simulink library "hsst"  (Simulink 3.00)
undefined symbols (not defined in the file or in its folder): Final, l, m3, s, to
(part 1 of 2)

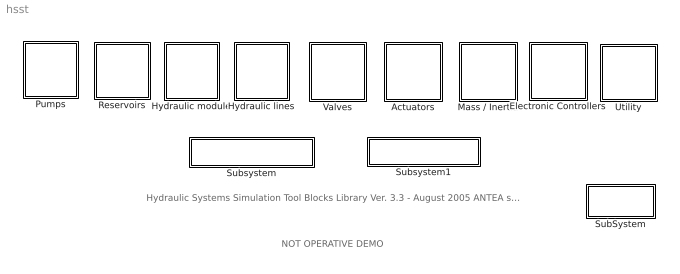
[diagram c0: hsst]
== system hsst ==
  note: Hydraulic Systems Simulation Tool Blocks Library Ver. 3.3 - August 2005 ANTEA s.a.s.
  note: NOT OPERATIVE DEMO
  Actuators : Subsystem
  Electronic Controllers : Subsystem
  Hydraulic lines : Subsystem
  Hydraulic module : Subsystem
  Mass / Inertia : Subsystem
  Pumps : Subsystem
  Reservoirs : Subsystem
  SubSystem : Subsystem
  Subsystem : Subsystem  StartFcn=Start_r
  Subsystem1 : Subsystem
  Utility : Subsystem
  Valves : Subsystem

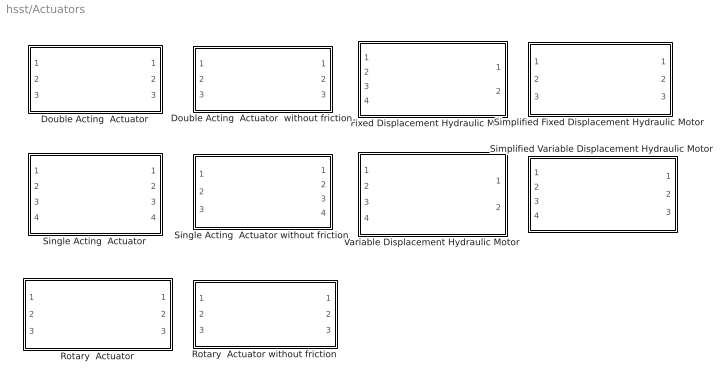
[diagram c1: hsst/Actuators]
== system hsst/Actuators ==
  Double Acting  Actuator : Subsystem  mask{Ai=, Au=, X_s=[0 0], m=, V0_out=1e-15, V0_in=1e-15, F0=, K=, C=, c_leak=, Fs=, Fd=}
      mask prompts: Ai "Piston Input Area [m2]"; Au "Piston Output Area [m2]"; X_s "Piston Maximum Stroke [m]"; m "Piston Mass [kg]"; V0_out "Piston Outlet Lost Volume [m3]"; V0_in "Piston Inlet Lost Volume [m3]"; F0 "Piston Spring Preload [N]"; K "Piston Spring Stiffness [N/m]"; C "Piston Damping [N/(m/s)]"; c_leak "Piston leakage coefficient [(m3/s)/sqr(Pa)]"; Fs "Static Friction Force [N]"; Fd "Dynamic Friction Force [N]"
      mask init:
      | global beta
  Double Acting  Actuator  without friction : Subsystem  mask{Ai=, Au=, X_s=[0 0], m=, V0_out=1.e-15, V0_in=1.e-15, F0=0, K=0, C=0}
      mask prompts: Ai "Piston Input Area [m2]"; Au "Piston Output Area [m2]"; X_s "Piston Maximum Stroke [m]"; m "Piston Mass [kg]"; V0_out "Piston Outlet Lost Volume [m3]"; V0_in "Piston Inlet Lost Volume [m3]"; F0 "Piston Spring Preload [N]"; K "Piston Spring Stiffness [N/m]"; C "Piston Damping [N/(m/s)]"
      mask init:
      | global beta
  Fixed Displacement Hydraulic Motor : Subsystem  mask(Hydraulic motor){Ds=0, Im=0, V0_out=0, Cm=0, cfug=0, c_leak=0, Ploss=0, Cf=0, rkm=0, Ts=0, Td=0}
      mask prompts: Ds "Displacement [cc/rev]"; Im "Total Motor Inertia [kg*m2]"; V0_out "Hydraulic line volume [m3]"; Cm "Actuator Internal Damping [Nm/(rad/s)]"; cfug "Interport Leakage coeff. [(m3/s)/Pa]"; c_leak "Case Drain Leakage Coef. [(m3/s)/Pa]"; Ploss "Ploss (Help for definition)"; Cf "Cf (Help for definition)"; rkm "rkm (Help for definition)"; Ts "Static FrictionTorque [Nm]"; Td "Dynamic Friction Torque [Nm]"
      mask init:
      | global beta
      | D = Ds/1e6;
      | V0_in = V0_out;
  Rotary  Actuator : Subsystem  mask(Rotary Actuator){Air=0, X_s=[0 0], m=0, V0_out=1e-15, F0=0, K=0, C=0, c_leak=0, Fs=0, Fd=0}
      mask prompts: Air "Displacement [cc/rev]"; X_s "Actuator Maximum Stroke [rad]"; m "Total Actuator Inertia [kg*m2]"; V0_out "Minimum Hydraulic Volume [m3]"; F0 "Actuator Spring Preload [Nm]"; K "Actuator Spring Stiffness [Nm/rad]"; C "Actuator Internal Damping [Nm/(rad/s)]"; c_leak "Actuator Internal Leakage Coefficient [(m3/s)/sqr(Pa)]"; Fs "Static Friction Force [N]"; Fd "Dynamic Friction Force [N]"
      mask init:
      | global beta
      | 
      | Ai = Air*1.e-6/6.2831853;
      | V0_in = V0_out;
      | Au = Ai;
  Rotary  Actuator without friction : Subsystem  mask(Rotary Actuator){Air=0, X_s=[0 0], m=0, V0_out=1e-15, F0=0, K=0, C=0}
      mask prompts: Air "Displacement [cc/rev]"; X_s "Actuator Maximum Stroke [rad]"; m "Total Actuator Inertia [kg*m2]"; V0_out "Minimum Hydraulic Volume [m3]"; F0 "Actuator Spring Preload [Nm]"; K "Actuator Spring Stiffness [Nm/rad]"; C "Actuator Internal Damping [Nm/(rad/s)]"
      mask init:
      | global beta
      | 
      | Ai = Air*1.e-6/6.2831853;
      | V0_in = V0_out;
      | Au = Ai;
  Simplified Fixed Displacement Hydraulic Motor : Subsystem  mask(Hydraulic motor){Ds=0, Im=0, V0_out=0, Cm=0, etav=0, etam=0}
      mask prompts: Ds "Displacement [cc/rev]"; Im "Total Motor Inertia [kg*m2]"; V0_out "Hydraulic line volume [m3]"; Cm "Actuator Internal Damping [Nm/(rad/s)]"; etav "Volumetric efficiency [-]"; etam "Mechanical  efficiency [-]"
      mask init:
      | global beta
      | D = Ds/1e6;
      | V0_in = V0_out;
  Simplified Variable Displacement Hydraulic Motor : Subsystem  mask(Variable diplacement hydraulic motor ){Ds_mx=0, Ds_mn=0, Im=0, V0_out=0, Cm=0, etav=0, etam=0}
      mask prompts: Ds_mx "Maximum Displacement [cc/rev]"; Ds_mn "Minimum Displacement [cc/rev]"; Im "Total Motor Inertia [kg*m2]"; V0_out "Hydraulic line volume [m3]"; Cm "Actuator Internal Damping [Nm/(rad/s)]"; etav "Volumetric efficiency [-]"; etam "Mechanical  efficiency [-]"
      mask init:
      | global beta
      | D_mx = Ds_mx/1e6;
      | D_mn = Ds_mn/1e6;
      | V0_in = V0_out;
  Single Acting  Actuator : Subsystem  mask(Single Acting Actuator){Ai=, Au=, X_s=[ ], m=, V0_in=1e-15, V0_out=1e-15, F0=, K=, C=, Fd=, Fs=}
      mask prompts: Ai "Piston Controlled Pressure Area [m2]"; Au "Piston Uncontrolled pressure Area [m2]"; X_s "Piston Maximum Stroke [m]"; m "Total Connected Mass [kg]"; V0_in "Piston Controlled Side Lost Volume [m3]"; V0_out "Piston Uncontrolled Side Lost Volume [m3]"; F0 "Piston Spring Preload [N]"; K "Piston Spring Stiffness [N/m]"; C "Piston Damping [N/(m/s)]"; Fd "Dyn. friction"; Fs "Static friction"
      mask init:
      | global beta
  Single Acting  Actuator without friction : Subsystem  mask(Single Acting Actuator){Ai=, Au=, X_s=[ ], m=, V0_in=1e-15, V0_out=1e-15, F0=, K=, C=}
      mask prompts: Ai "Piston Controlled Pressure Area [m2]"; Au "Piston Uncontrolled pressure Area [m2]"; X_s "Piston Maximum Stroke [m]"; m "Total Connected Mass [kg]"; V0_in "Piston Controlled Side Lost Volume [m3]"; V0_out "Piston Uncontrolled Side Lost Volume [m3]"; F0 "Piston Spring Preload [N]"; K "Piston Spring Stiffness [N/m]"; C "Piston Damping [N/(m/s)]"
      mask init:
      | global beta
  Variable Displacement Hydraulic Motor : Subsystem  mask(Variable diplacement hydraulic motor ){Ds_mx=0, Ds_mn=0, Im=0, V0_out=0, Cm=0, cfug=0, c_leak=0, Ploss=0, Cf=0, rkm=0, Ts=0, Td=0}
      mask prompts: Ds_mx "Maximum Displacement [cc/rev]"; Ds_mn "Minimum Displacement [cc/rev]"; Im "Total Motor Inertia [kg*m2]"; V0_out "Hydraulic line volume [m3]"; Cm "Actuator Internal Damping [Nm/(rad/s)]"; cfug "Interport Leakage coeff. [(m3/s)/Pa]"; c_leak "Case Drain Leakage Coef. [(m3/s)/Pa]"; Ploss "Ploss (Help for definition)"; Cf "Cf (Help for definition)"; rkm "rkm (Help for definition)"; Ts "Static FrictionTorque [Nm]"; Td "Dynamic Friction Torque [Nm]"
      mask init:
      | global beta
      | D_mx = Ds_mx/1e6;
      | D_mn = Ds_mn/1e6;
      | V0_in = V0_out;

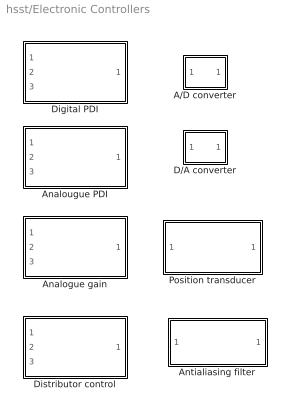
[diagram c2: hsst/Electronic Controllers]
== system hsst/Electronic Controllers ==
  A/D converter : Subsystem  mask(A/D){n_bit=, n_max=}
      mask prompts: n_bit "Number of bit (excluding the sign bit: saturation = +/- n° bit)"; n_max "Satuaration value  (output saturation at +/- this value)"
      mask init:
      | lsb=n_max/2^n_bit;
  Analogue gain : Subsystem  mask(Analog controller){Gp=, H=, p_opm=}
      mask prompts: Gp "Proportional gain"; H "Feedback gain"; p_opm "Minimum Operative Pressure [MPa]"
      mask init:
      | p_op=p_opm*1.e6;
  Analougue PDI : Subsystem  mask(Analuogue PDI controller){Gp=[ ], Gi=[ ], Gd=[ ], tau=, Ls=[ ], Ls_1=[-Inf Inf], i_i_max=[-Inf Inf], H=, p_opm=, max_cp=Inf, max_cm=-Inf}
      mask prompts: Gp "Proportional gain (2 values: [- +])"; Gi "Integrative gain (2 values: [- +])"; Gd "Derivative gain (2 values: [- +])"; tau "First order filter constant [s]"; Ls "Integrator threshold (2 values)"; Ls_1 "Integrator band limit (2 values)"; i_i_max "Integrator current saturation [mA] (2 val)"; H "Feedback gain"; p_opm "Minimum Operative Pressure [MPa]"; max_cp "max curr"; max_cm "min curr"
      mask help: Digital PDI controller
      mask init:
      | % i_i_min=-i_i_max;
      | % Li=-Ls;
      | % Li_1=-Ls_1;
      | p_op=p_opm*1.e6;
  Antialiasing filter : Subsystem  mask(Antialiasing filter){fr=, zi=}
      mask prompts: fr "Undumped natural frequency [Hz]"; zi "Damping factor"
      mask init:
      | sig=2*pi*fr;
  D/A converter : Subsystem  mask(A/D){n_bit=, n_max=}
      mask prompts: n_bit "Number of bit (excluding the sign bit: saturation = +/- n° bit)"; n_max "Satuaration value  (output saturation at +/- this value)"
      mask init:
      | lsb=n_max/2^n_bit;
  Digital PDI : Subsystem  mask(PDI controller){Ts=, Tc=, Gp=[ ], Gi=[ ], Gd=[ ], tau=, Ls=[ ], Ls_1=[-Inf Inf], i_i_max=[-Inf Inf], H=, p_opm=, max_cp=Inf, max_cm=-Inf}
      mask prompts: Ts "Sampling time [s]"; Tc "Calculation time [s]"; Gp "Proportional gain (2 values: [- +])"; Gi "Integrative gain (2 values: [- +])"; Gd "Derivative gain (2 values: [- +])"; tau "First order filter constant [s]"; Ls "Integrator threshold (2 values)"; Ls_1 "Integrator band limit (2 values)"; i_i_max "Integrator current saturation [mA] (2 val)"; H "Feedback gain"; p_opm "Minimum Operative Pressure [MPa]"; max_cp "max curr"; max_cm "min curr"
      mask help: Digital PDI controller
      mask init:
      | % i_i_min=-i_i_max;
      | % Li=-Ls;
      | % Li_1=-Ls_1;
      | p_op=p_opm*1.e6;
  Distributor control : Subsystem  mask(Distributor controller){c_mx=, H=, p_opm=}
      mask prompts: c_mx "Maximum current"; H "Feedback gain"; p_opm "Minimum Operative Pressure [MPa]"
      mask init:
      | p_op=p_opm*1.e6;
  Position transducer : Subsystem  mask{bksl=}
      mask prompts: bksl "Position transducer backlash [actuator position unit]"

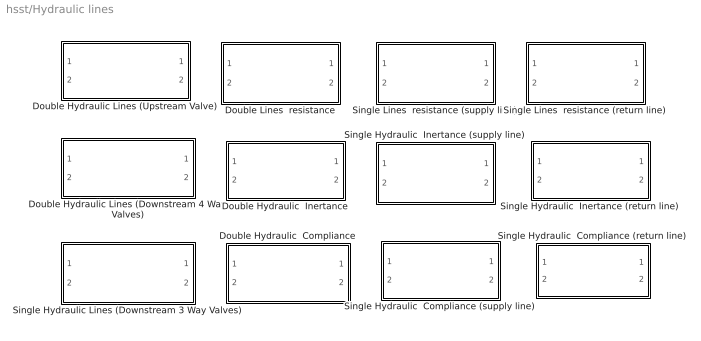
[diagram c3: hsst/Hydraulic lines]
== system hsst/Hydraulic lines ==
  Double Hydraulic  Compliance : Subsystem  mask(Double Hydraulic Compliance){C1=, C2=}
      mask prompts: C1 "Line 1 hydraulic compliance [m5/N]"; C2 "Line 2 hydraulic compliance [m5/N]"
  Double Hydraulic  Inertance : Subsystem  mask(Double Hydraulic Lines){rl1=, rl2=, rq1=, rq2=, L1=, L2=}
      mask prompts: rl1 "Line 1 linear resistance coefficient [Pa s/m3]"; rl2 "Line 2 linear resistance coefficient [Pa s/m3]"; rq1 "Line 1 quadratic resistance coefficient [Pa s2/m6]"; rq2 "Line 2 quadratic resistance coefficient [Pa s2/m6]"; L1 "Line 1 inertance [kg/m4]"; L2 "Line 2 inertance [kg/m4]"
  Double Hydraulic Lines (Downstream 4 Way Valves) : Subsystem  mask(Hydraulic Line){rl1=, rl2=, rq1=, rq2=, ll1=, ll2=, a1=, a2=}
      mask prompts: rl1 "Line 1 linear resistance coefficient [Pa s/m3]"; rl2 "Line 2 linear resistance coefficient [Pa s/m3]"; rq1 "Line 1 quadratic resistance coefficient [Pa s2/m6]"; rq2 "Line 2 quadratic resistance coefficient [Pa s2/m6]"; ll1 "Line 1 length [m]"; ll2 "Line 2  length [m]"; a1 "Line 1 section area [m2]"; a2 "Line 2 section area [m2]"
      mask init:
      | global rho
      | global beta
      | L1 = rho*ll1/a1;
      | L2 = rho*ll2/a2;
  Double Hydraulic Lines (Upstream Valve) : Subsystem  mask(Hydraulic Line){rl1=, rl2=, rq1=, rq2=, ll1=, ll2=, a1=, a2=}
      mask prompts: rl1 "Line 1 linear resistance coefficient [Pa s/m3]"; rl2 "Line 2 linear resistance coefficient [Pa s/m3]"; rq1 "Line 1 quadratic resistance coefficient [Pa s2/m6]"; rq2 "Line 2 quadratic resistance coefficient [Pa s2/m6]"; ll1 "Line 1 length [m]"; ll2 "Line 2  length [m]"; a1 "Line 1 section area [m2]"; a2 "Line 2 section area [m2]"
      mask init:
      | global rho
      | global beta
      | L1 = rho*ll1/a1;
      | L2 = rho*ll2/a2;
  Double Lines  resistance : Subsystem  mask(Lines resistance){rq1=, rl1=, rq2=, rl2=}
      mask prompts: rq1 "Line 1 quadratic resistance [Pa/(m6/s2)]"; rl1 "Line 1 linear resistance [Pa/(m3/s)]"; rq2 "Line 2 quadratic resistance [Pa/(m6/s2)]"; rl2 "Line 2 linear resistance [Pa/(m3/s)]"
      mask init:
      | global rho
      | global mu
      | q_min=.01/60000;
  Single Hydraulic  Compliance (return line) : Subsystem  mask(Single Hydraulic Compliance){C1=}
      mask prompts: C1 "Hydraulic compliance [m5/N]"
  Single Hydraulic  Compliance (supply line) : Subsystem  mask(Single Hydraulic Compliance){C1=}
      mask prompts: C1 "Hydraulic compliance [m5/N]"
  Single Hydraulic  Inertance (return line) : Subsystem  mask(Single Hydraulic Lines){rl1=, rq1=, L1=}
      mask prompts: rl1 "Linear resistance coefficient [Pa s/m3]"; rq1 "Quadratic resistance coefficient [Pa s2/m6]"; L1 "Inertance [kg/m4]"
  Single Hydraulic  Inertance (supply line) : Subsystem  mask(Single Hydraulic Lines){rl1=, rq1=, L1=}
      mask prompts: rl1 "Linear resistance coefficient [Pa s/m3]"; rq1 "Quadratic resistance coefficient [Pa s2/m6]"; L1 "Inertance [kg/m4]"
  Single Hydraulic Lines (Downstream 3 Way Valves) : Subsystem  mask(Hydraulic Line){rl1=, rq1=, ll1=, a1=}
      mask prompts: rl1 "Line linear resistance coefficient [Pa s/m3]"; rq1 "Line  quadratic resistance coefficient [Pa s2/m6]"; ll1 "Line  length [m]"; a1 "Line section area [m2]"
      mask init:
      | global rho
      | global beta
      | L1 = rho*ll1/a1;
  Single Lines  resistance (return line) : Subsystem  mask(Lines resistance){rq1=, rl1=}
      mask prompts: rq1 "Line 1 quadratic resistance [Pa/(m6/s2)]"; rl1 "Line 1 linear resistance [Pa/(m3/s)]"
      mask init:
      | global rho
      | global mu
      | q_min=.01/60000;
  Single Lines  resistance (supply line) : Subsystem  mask(Lines resistance){rq1=, rl1=}
      mask prompts: rq1 "Line 1 quadratic resistance [Pa/(m6/s2)]"; rl1 "Line 1 linear resistance [Pa/(m3/s)]"
      mask init:
      | global rho
      | global mu
      | q_min=.01/60000;

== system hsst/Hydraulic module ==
  Accumulator : Subsystem  mask(Accumulator){ti=20, Tp=20, cv=742, h_gas=.2, hy_compl=4e-14, vi=, pp=, r_gas=287}
      mask prompts: ti "Initial liquid temperature [°C]"; Tp "Precharge temperature [°C]"; cv "Gas specific heat (cv) [J/(K kg)]"; h_gas "Heat exchange coefficient [W/K]"; hy_compl "Hydraulic compliance (with acc. discharged)[m5/N]"; vi "Precharge volume [l]"; pp "Precharge pressure [MPa]"; r_gas "Gas constant [J/(kg K)]"
      mask help: Model of a hydraulic accumulator.
      mask init:
      | global rho
      | 
      | t_liq = ti+273;
      | t_pr = Tp+273;
      | T0 = t_liq;
      | P0 = pp*1e6;
      | v0=vi/1000;
      | m_gas=P0*v0/(r_gas*t_pr);
      | P0 = pp*1e6*T0/t_pr;
  Accumulator (Adiabatic) : Subsystem  mask(Accumulator){hy_compl=4e-14, vi=, pp=, gamma=1.4}
      mask prompts: hy_compl "Hydraulic compliance (with acc. discharged)[m5/N]"; vi "Precharge volume [l]"; pp "Precharge pressure [MPa]"; gamma "Polytropic coeficient [-)]"
      mask help: Model of a hydraulic accumulator.
      mask init:
      | global rho
      | 
      | P0 = pp*1e6;
      | v0=vi/1000;
  Filter : Subsystem  mask(Filter){r_filter=, dp=}
      mask prompts: r_filter "Filter pressure drop coefficient [Pa s2/m6]"; dp "Constant  pressure drop [Pa]"
  Pressure relief : Subsystem  mask(Relief Valve){Pi=, Pmx=, flw=, cd=0.61}
      mask prompts: Pi "Breacking pressure [MPa]"; Pmx "Full open pressure   [MPa]"; flw "Maximum flow [l/min]"; cd "Discharge coefficient"
      mask init:
      | global rho
      | p_max=Pi*1e6;
      | p_lim_mx=Pmx*1e6;
      | a_f_rho=flw/60000/cd*sqrt(1/(2*p_lim_mx));
  Pressure reducer : Subsystem

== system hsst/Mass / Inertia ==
  Stifness & Mass : Subsystem  mask(Mass & stiffness){m2=, k_sha=, c_sha=, X_max=, X_min=, k_spr2=, F00=, c2=, Fs1=, Fd1=, rapp=}
      mask prompts: m2 "Total mass downstream ratio [kg]"; k_sha "Connection Spring Stiffness downstream ratio [N/m]"; c_sha "Connection Spring Damping coeff. downstream ratio [Ns/m]"; X_max "Maximum positive stroke downstream ratio [m]"; X_min "Maximum negative stroke downstream ratio [m]"; k_spr2 "External Spring Stiffness downstream ratio [N/m]"; F00 "External Spring Preload downstream ratio [N]"; c2 "External Damping coeff. downstream ratio [N s/m]"; Fs1 "Static friction force downstream ratio [N]"; Fd1 "Dynamic friction force downstream ratio [N]"; rapp "Transmis. ratio (output position  over input [-])"
      mask init:
      | X_max2 = X_max /rapp;
      | X_min2 = X_min /rapp:
      | Fd = Fd1*rapp;
      | Fs = Fs1*rapp;
  "Stifness & Mass withiout friction " : Subsystem  mask(Mass & stiffness){m2=, k_sha=, c_sha=, X_max=, X_min=, k_spr2=, F00=, c2=, rapp=}
      mask prompts: m2 "Total mass downstream ratio [kg]"; k_sha "Connection Spring Stiffness downstream ratio [N/m]"; c_sha "Connection Spring Damping coeff. downstream ratio [Ns/m]"; X_max "Maximum positive stroke downstream ratio [m]"; X_min "Maximum negative stroke downstream ratio [m]"; k_spr2 "External Spring Stiffness downstream ratio [N/m]"; F00 "External Spring Preload downstream ratio [N]"; c2 "External Damping coeff. downstream ratio [N s/m]"; rapp "Transmis. ratio (output position  over input [-])"
      mask init:
      | X_max2 = X_max /rapp;
      | X_min2 = X_min /rapp:
  Stifness & Mass  with non linear ratio : Subsystem  mask(Mass & stiffness){m2=, k_sha=, c_sha=, X_max2=, X_min2=, k_spr2=, F00=, c2=, Fs=, Fd=, rapp=[1 0 0 0 0]}
      mask prompts: m2 "Total mass downstream ratio [kg]"; k_sha "Connection Spring Stiffness downstream ratio [N/m]"; c_sha "Connection Spring Damping coeff. downstream ratio [Ns/m]"; X_max2 "Maximum positive stroke upstream ratio [m]"; X_min2 "Maximum negative stroke upstream ratio [m]"; k_spr2 "External Spring Stiffness downstream ratio [N/m]"; F00 "External Spring Preload downstream ratio [N]"; c2 "External Damping coeff. downstream ratio [N s/m]"; Fs "Static friction force downstream ratio [N]"; Fd "Dynamic friction force downstream ratio [N]"; rapp "Transmis. ratio: 5 exponents of polynom. (ratio vs position [m])"
      mask init:
      | deltateta=(X_max2 - X_min2)/100;
  Stifness & Mass  with non linear ratio without friction : Subsystem  mask(Mass & stiffness){m2=, k_sha=, c_sha=, X_max2=, X_min2=, k_spr2=, F00=, c2=, rapp=[1 0 0 0 0]}
      mask prompts: m2 "Total mass downstream ratio [kg]"; k_sha "Connection Spring Stiffness downstream ratio [N/m]"; c_sha "Connection Spring Damping coeff. downstream ratio [Ns/m]"; X_max2 "Maximum positive stroke upstream ratio [m]"; X_min2 "Maximum negative stroke upstream ratio [m]"; k_spr2 "External Spring Stiffness downstream ratio [N/m]"; F00 "External Spring Preload downstream ratio [N]"; c2 "External Damping coeff. downstream ratio [N s/m]"; rapp "Transmis. ratio: 5 exponents of polynom. (ratio vs position [m])"
      mask init:
      | deltateta=(X_max2 - X_min2)/100;
  Stifness & Rotating Mass : Subsystem  mask(Rotating Mass & Stiffness ){m2=, k_sha=, c_sha=, X_max=, X_min=, k_spr2=, F00=, c2=, Fs1=, Fd1=, rapp=}
      mask prompts: m2 "Total inertia downstream ratio [kg*m2]"; k_sha "Connection Spring Stiffness downstream ratio [Nm/rad]"; c_sha "Connection Spring Damping coeff. downstream ratio [Nms/rad]"; X_max "Maximum positive stroke downstream ratio [rad]"; X_min "Maximum negative stroke downstream ratio [rad]"; k_spr2 "External Spring Stiffness downstream ratio [Nm/rad]"; F00 "External Spring Preload downstream ratio [Nm]"; c2 "External Damping coeff. downstream ratio [Nm s/rad]"; Fs1 "Static friction torque  downstream ratio [Nm]"; Fd1 "Dynamic friction torque  downstream ratio [Nm]"; rapp "Transmis. ratio (output position over input position) [-]"
      mask init:
      | X_max2 = X_max /rapp;
      | X_min2 = X_min /rapp:
      | Fs = Fs1*rapp;
      | Fd =Fd1*rapp;
  Stifness & Rotating Mass without friction : Subsystem  mask(Rotating Mass & Stiffness ){m2=, k_sha=, c_sha=, X_max=, X_min=, k_spr2=, F00=, c2=, rapp=}
      mask prompts: m2 "Total inertia downstream ratio [kg*m2]"; k_sha "Connection Spring Stiffness downstream ratio [Nm/rad]"; c_sha "Connection Spring Damping coeff. downstream ratio [Nms/rad]"; X_max "Maximum positive stroke downstream ratio [rad]"; X_min "Maximum negative stroke downstream ratio [rad]"; k_spr2 "External Spring Stiffness downstream ratio [Nm/rad]"; F00 "External Spring Preload downstream ratio [Nm]"; c2 "External Damping coeff. downstream ratio [Nm s/rad]"; rapp "Transmis. ratio (output position over input position) [-]"
      mask init:
      | X_max2 = X_max /rapp;
      | X_min2 = X_min /rapp:
  Stifness & Rotating Mass  with non linear ratio : Subsystem  mask(Rotating Mass & stiffness){m2=, k_sha=, c_sha=, X_max2=, X_min2=, k_spr2=, F00=, c2=, Fs=, Fd=, rapp=[1 0 0 0 0]}
      mask prompts: m2 "Total inertia downstream ratio [kg*m2]"; k_sha "Connection Spring Stiffness downstream ratio [Nm/rad]"; c_sha "Connection Spring Damping coeff. downstream ratio [Nms/rad]"; X_max2 "Maximum positive stroke upstream ratio [rad]"; X_min2 "Maximum negative stroke upstream ratio [rad]"; k_spr2 "External Spring Stiffness downstream ratio [Nm/rad]"; F00 "External Spring Preload downstream ratio [Nm]"; c2 "External Damping coeff. downstream ratio [Nm s/rad]"; Fs "Static friction torque  downstream ratio [Nm]"; Fd "Dynamic friction torque  downstream ratio [Nm]"; rapp "Transmis. ratio: 5 exponents of polynom. (ratio vs position [rad])"
      mask init:
      | deltateta=(X_max2 - X_min2)/100;
  Stifness & Rotating Mass  with non linear ratio without friction : Subsystem  mask(Rotating Mass & stiffness){m2=, k_sha=, c_sha=, X_max2=, X_min2=, k_spr2=, F00=, c2=, rapp=[1 0 0 0 0]}
      mask prompts: m2 "Total inertia downstream ratio [kg*m2]"; k_sha "Connection Spring Stiffness downstream ratio [Nm/rad]"; c_sha "Connection Spring Damping coeff. downstream ratio [Nms/rad]"; X_max2 "Maximum positive stroke upstream ratio [rad]"; X_min2 "Maximum negative stroke upstream ratio [rad]"; k_spr2 "External Spring Stiffness downstream ratio [Nm/rad]"; F00 "External Spring Preload downstream ratio [Nm]"; c2 "External Damping coeff. downstream ratio [Nm s/rad]"; rapp "Transmis. ratio: 5 exponents of polynom. (ratio vs position [rad])"
      mask init:
      | deltateta=(X_max2 - X_min2)/100;

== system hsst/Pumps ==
  1 Fixed displacement pump : Subsystem  mask(Fixed displacement pump){delta=, eta_m=, eta_vol=, rho_e=, mu_e=, beta_e=}
      mask prompts: delta "Pump displacement [cc/rev]"; eta_m "Mechanical efficiency"; eta_vol "Volumetric efficiency"; rho_e "Fluid density [kg/m3]"; mu_e "Fluid viscosity [kg/ms]"; beta_e "Bulk modulus [MPa]"
      mask help: Model of a fixed displacement pump. Input: angular speed [rpm] output: supplied flow [m3/s] The internal leakage value [m3/s] is stored into the global variable 'pump_leak', that can be read by a 'From' block
      mask init:
      | global rho
      | global mu
      | global beta
      | rho=rho_e;
      | mu=mu_e;
      | beta=beta_e*1e6;
      | dlt=delta*1e-6/60;
  1 Hydraulic Supply : Subsystem  mask(Variable Displacement Pump){Ps=, Pr=, rho_e=, mu_e=, beta_e=}
      mask prompts: Ps "System Supply Pressure [MPa]"; Pr "System Return Pressure [MPa]"; rho_e "Fluid density [kg/m3]"; mu_e "Fluid viscosity [kg/ms]"; beta_e "Bulk modulus [MPa]"
      mask help: Model of a variable displacement pump.
      mask init:
      | global rho
      | global mu
      | global beta
      | rho=rho_e;
      | mu=mu_e;
      | beta=beta_e*1e6;
      | P_s = Ps*1.e6;
      | P_r = Pr*1.e6;
  1 Variable displacement pump : Subsystem  mask(Variable Displacement Pump){deltax=, deltamn=, pm_min=, pm_max=, tau=, eta_m=, eta_vol=, rho_e=, mu_e=, beta_e=}
      mask prompts: deltax "Pump max displacement [cc/rev]"; deltamn "Pump min displacement [cc/rev]"; pm_min "Minimum compensation pressure [MPa]"; pm_max "Maximum compensation pressure [MPa]"; tau "Compensator time constant [s]"; eta_m "Mechanical efficiency"; eta_vol "Volumetric efficiency"; rho_e "Fluid density [kg/m3]"; mu_e "Fluid viscosity [kg/ms]"; beta_e "Bulk modulus [MPa]"
      mask help: Model of a variable displacement pump.
      mask init:
      | global rho
      | global mu
      | global beta
      | rho=rho_e;
      | mu=mu_e;
      | beta=beta_e*1e6;
      | dlt_max=deltax*1e-6/60;
      | dlt_min=deltamn*1e-6/60;
      | p_max = pm_max*1.e6;
      | p_min = pm_min*1.e6;

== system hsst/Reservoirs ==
  Atmosferic reservoir : Subsystem  mask(Atmosferic reservoir){v_cc=}
      mask prompts: v_cc "Initial fluid volume [cc]"
      mask help: Model of an atmosferic reservoir; Input: 1 - Return flows from the systems (is a vector) [m3/s] 2 - Pump flow [m3/s] 3 - Relief valve flow [m3/s] 4 - Single Acting Actuators flow of the uncontrolled pressure side Output: Reservoir volume [cc]
      mask init:
      | v_reser=v_cc/1e6;
  Pressurised reservoir : Subsystem  mask(Pressurised Reservoir){v_cc=, a_hp=, a_lp=, k_spr_res=, f0_res=}
      mask prompts: v_cc "Initial fluid volume [cc]"; a_hp "High pressure side area [m2]"; a_lp "Low pressure side area  [m2]"; k_spr_res "Spring stiffness [N/m]"; f0_res "Spring preload [N]"
      mask help: Model of a pressurised reservoir;
      mask init:
      | v_reser=v_cc/1e6;

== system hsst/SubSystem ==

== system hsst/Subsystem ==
  Init : Subsystem  mask(Initialisation){Name_in=Final, Name_fin=Final, Ch=Unitialised Condition, Sav=off}
      mask prompts: Name_in "Initial state File Name"; Name_fin "Final state File Name"; Ch "Start from"; Sav "Save Current States to File"
      mask init:
      | global nome_f
      | global nome_i

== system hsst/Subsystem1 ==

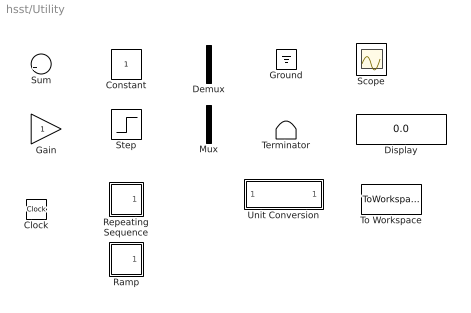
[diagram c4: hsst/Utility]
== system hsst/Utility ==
  Clock : Clock
  Constant : Constant  Value=1
  Demux : Demux  Outputs=2
  Display : Display
  Gain : Gain  Gain=1  SaturateOnIntegerOverflow=on
  Ground : Ground
  Mux : Mux  Inputs=2
  Ramp : Subsystem  mask(Ramp){slope=1, start=0, X0=0}
      mask prompts: start "Start time:"; X0 "Initial output:"
      mask help: ramp
  Repeating Sequence : Subsystem  mask(Repeating table){rep_seq_t=[0 2], rep_seq_y=[0 2]}
      mask prompts: rep_seq_t "Time values:"; rep_seq_y "Output values:"
      mask help: Repeating table.
      mask init:
      | period = max(rep_seq_t);
  Scope : Scope
  Step : Step  Time=1  Before=0  After=1  SampleTime=0
  Sum : Sum  Inputs=|++  SaturateOnIntegerOverflow=on
  Terminator : Terminator
  To Workspace : ToWorkspace  VariableName=simout  SampleTime=-1  SaveFormat=Matrix
  Unit Conversion : Subsystem  mask(Unit conversion){Ch=m3/s to l/min}
      mask prompts: Ch "Conversion type"
      mask init:
      | if Ch==1
      |   gain = 6e4;
      |  dsp = 'm3/s to l/min';
      | end
      | if Ch==2
      |   gain = 6.102e4;
      |   dsp = 'm3/s to cis';
      | end
      | if Ch==3
      |   gain = 15852;
      |   dsp = 'm3/s to gpm';
      | end
      | if Ch==4
      |   gain = 1e-6;
      |   dsp = 'Pa to MPa';
      | end
      | if Ch==5
      |   gain = 1.4503e-4;
      |   dsp = 'Pa to psi';
      | end
      | if Ch==6
      |   gain = 1000;
      |   dsp = 'm to mm';
      | end
      | if Ch==7
      |   gain = 39.37;
      |   dsp = 'm to in';
      | end
      | if Ch==8
      |   gain = 180/pi;
      |   dsp = 'rad to deg';
      | end
      | if Ch==9
      |   gain = 30/pi;
      |   dsp = 'rad/s to rpm';
      | end
      | 
      | gain = 1;

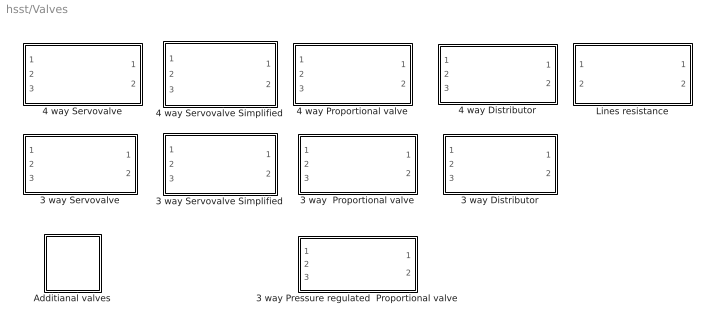
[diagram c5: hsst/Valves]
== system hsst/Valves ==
  3 way  Proportional valve : Subsystem
  3 way Distributor : Subsystem  mask(3 way distributor){xm=, cc1=, ta=, Os=, Or=, hh=, ww=, ccd=}
      mask prompts: xm "Spool Maximum Displacement [m]"; cc1 "Electrical Gain [m/mA]"; ta "Time response [s]"; Os "Overlap Supply [m]"; Or "Overlap Return [m]"; hh "Radial Clearance [m]"; ww "Port Width [m]"; ccd "Discharge Coefficient [-]"
  3 way Pressure regulated  Proportional valve : Subsystem
  3 way Servovalve : Subsystem
  3 way Servovalve Simplified : Subsystem  mask(Simplified 3 way servovalve){i_max=, n_flow=, n_dp=, Ovr=, kf=, fr=, Zv=}
      mask prompts: i_max "Nominal current [mA]"; n_flow "Nominal flow [l/min]"; n_dp "Nominal pressure drop [MPa]"; Ovr "Overlap (current) [mA]"; kf "First stage flow coefficient [m3/s/sqrt(Pa)]"; fr "Valve Resonance Frequency [Hz]"; Zv "Valve Damping Factor [-]"
      mask init:
      | flow=n_flow/6e4;
      | dp=n_dp*1e6;
      | k_flow = flow/(i_max*sqrt(dp));
      | Wv=fr*2*pi;
  4 way Distributor : Subsystem  mask(4 way distributor){xm=, cc1=, ta=, Os=, Or=, hh=, ww=, ccd=}
      mask prompts: xm "Spool Maximum Displacement [m]"; cc1 "Electrical Gain [m/mA]"; ta "Time response [s]"; Os "Overlap Supply [m]"; Or "Overlap Return [m]"; hh "Radial Clearance [m]"; ww "Port Width [m]"; ccd "Discharge Coefficient [-]"
  4 way Proportional valve : Subsystem
  4 way Servovalve : Subsystem
  4 way Servovalve Simplified : Subsystem  mask(Simplified 4 way servovalve){i_max=, n_flow=, n_dp=, Ovr=, kf=, fr=, Zv=}
      mask prompts: i_max "Nominal current [mA]"; n_flow "Nominal flow [l/min]"; n_dp "Nominal pressure drop [MPa]"; Ovr "Overlap (current) [mA]"; kf "First stage flow coefficient [m3/s/sqrt(Pa)]"; fr "Valve Resonance Frequency [Hz]"; Zv "Valve Damping Factor [-]"
      mask init:
      | flow=n_flow/6e4;
      | dp=n_dp*1e6;
      | k_flow = flow/(i_max*sqrt(2*dp));
      | Wv=fr*2*pi;
  Additianal valves : Subsystem
  Lines resistance : Subsystem  mask(Lines resistance){rq1=, rl1=, rq2=, rl2=}
      mask prompts: rq1 "Line 1 quadratic resistance [Pa/(m6/s2)]"; rl1 "Line 1 linear resistance [Pa/(m3/s)]"; rq2 "Line 2 quadratic resistance [Pa/(m6/s2)]"; rl2 "Line 2 linear resistance [Pa/(m3/s)]"
      mask init:
      | global rho
      | global mu
      | q_min=.01/60000;

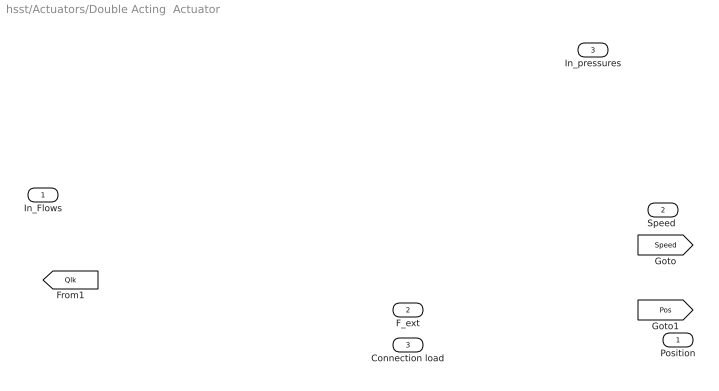
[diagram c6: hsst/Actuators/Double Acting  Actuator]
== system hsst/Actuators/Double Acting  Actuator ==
  In_Flows : Inport  Port=1  PortWidth=-1  SampleTime=-1  DataType=auto
  F_ext : Inport  Port=2  PortWidth=-1  SampleTime=-1  DataType=auto
  Connection load : Inport  Port=3  PortWidth=-1  SampleTime=-1  DataType=auto
  Position : Outport  Port=1
  "Speed " : Outport  Port=2
  In_pressures : Outport  Port=3
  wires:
  In_Flows/1 -> ?
  F_ext/1 -> ?
  Connection load/1 -> ?

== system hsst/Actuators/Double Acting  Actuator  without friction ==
  In_Flows : Inport  Port=1  PortWidth=-1  SampleTime=-1  DataType=auto
  F_ext : Inport  Port=2  PortWidth=-1  SampleTime=-1  DataType=auto
  Connection load : Inport  Port=3  PortWidth=-1  SampleTime=-1  DataType=auto
  Position : Outport  Port=1
  Speed : Outport  Port=2
  In_Pressures : Outport  Port=3
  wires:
  ? -> Position/1, [Pos]
  In_Flows/1 -> ?
  ? -> [Speed], Speed/1

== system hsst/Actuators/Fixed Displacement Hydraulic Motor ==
  In_Flows : Inport  Port=1  PortWidth=-1  SampleTime=-1  DataType=auto
  T_ext : Inport  Port=2  PortWidth=-1  SampleTime=-1  DataType=auto
  System_Pressures : Inport  Port=3  PortWidth=-1  SampleTime=-1  DataType=auto
  Connection Torque : Inport  Port=4  PortWidth=-1  SampleTime=-1  DataType=auto
  Position : Outport  Port=1
  Speed : Outport  Port=2
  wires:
  In_Flows/1 -> ?
  ? -> Position/1
  Connection Torque/1 -> ?
  T_ext/1 -> ?
  ? -> [Speed], Speed/1

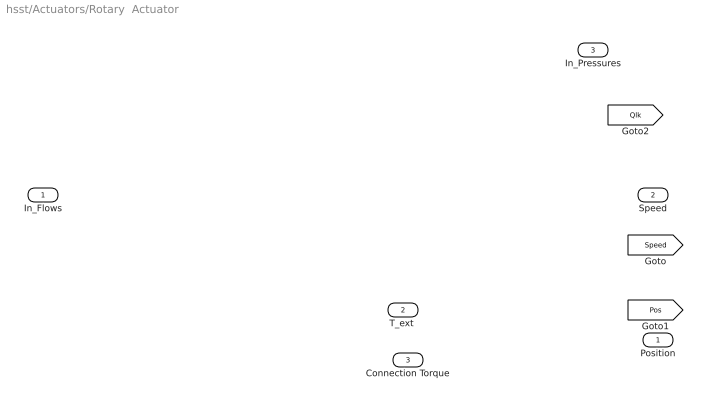
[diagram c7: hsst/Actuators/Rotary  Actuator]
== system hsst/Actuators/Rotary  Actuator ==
  In_Flows : Inport  Port=1  PortWidth=-1  SampleTime=-1  DataType=auto
  "T_ext " : Inport  Port=2  PortWidth=-1  SampleTime=-1  DataType=auto
  Connection Torque : Inport  Port=3  PortWidth=-1  SampleTime=-1  DataType=auto
  Position : Outport  Port=1
  Speed : Outport  Port=2
  In_Pressures : Outport  Port=3
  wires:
  ? -> [Qlk]
  ? -> Position/1, [Pos]
  Connection Torque/1 -> ?
  "T_ext "/1 -> ?
  ? -> [Speed], Speed/1

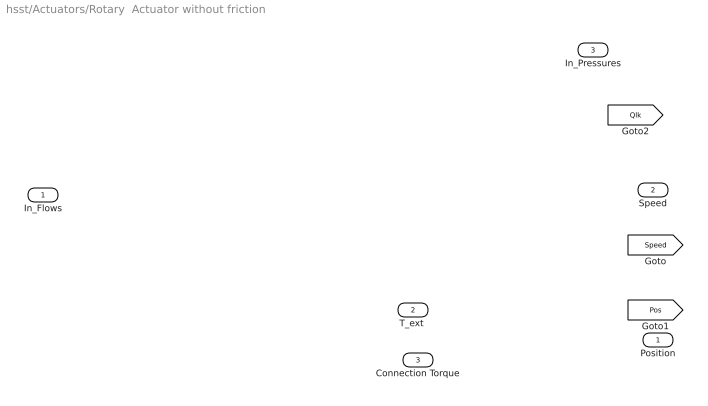
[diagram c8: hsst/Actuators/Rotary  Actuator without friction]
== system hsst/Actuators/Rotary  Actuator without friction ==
  In_Flows : Inport  Port=1  PortWidth=-1  SampleTime=-1  DataType=auto
  "T_ext " : Inport  Port=2  PortWidth=-1  SampleTime=-1  DataType=auto
  Connection Torque : Inport  Port=3  PortWidth=-1  SampleTime=-1  DataType=auto
  Position : Outport  Port=1
  Speed : Outport  Port=2
  In_Pressures : Outport  Port=3
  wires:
  In_Flows/1 -> ?
  ? -> [Pos], Position/1
  ? -> [Qlk]
  Connection Torque/1 -> ?
  "T_ext "/1 -> ?
  ? -> [Speed], Speed/1

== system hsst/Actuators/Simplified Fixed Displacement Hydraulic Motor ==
  In_Flows : Inport  Port=1  PortWidth=-1  SampleTime=-1  DataType=auto
  T_ext : Inport  Port=2  PortWidth=-1  SampleTime=-1  DataType=auto
  Connection Torque : Inport  Port=3  PortWidth=-1  SampleTime=-1  DataType=auto
  Position : Outport  Port=1
  In_Pressures : Outport  Port=2
  Speed : Outport  Port=3
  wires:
  ? -> Speed/1, [Speed]
  ? -> Position/1
  ? -> In_Pressures/1
  In_Flows/1 -> ?

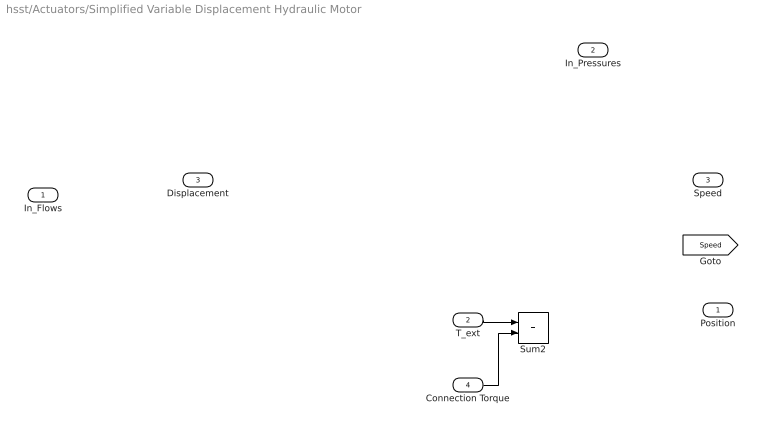
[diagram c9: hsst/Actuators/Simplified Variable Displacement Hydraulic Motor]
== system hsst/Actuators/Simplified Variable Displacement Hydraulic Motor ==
  In_Flows : Inport  Port=1  PortWidth=-1  SampleTime=-1  DataType=auto
  T_ext : Inport  Port=2  PortWidth=-1  SampleTime=-1  DataType=auto
  Displacement : Inport  Port=3  PortWidth=-1  SampleTime=-1  DataType=auto
  Connection Torque : Inport  Port=4  PortWidth=-1  SampleTime=-1  DataType=auto
  Sum2 : Sum  Inputs=++  SaturateOnIntegerOverflow=on
  Position : Outport  Port=1
  In_Pressures : Outport  Port=2
  Speed : Outport  Port=3
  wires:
  ? -> Speed/1, [Speed]
  T_ext/1 -> Sum2/1
  Sum2/1 -> ?
  Connection Torque/1 -> Sum2/2
  ? -> Position/1
  ? -> In_Pressures/1
  Displacement/1 -> ?

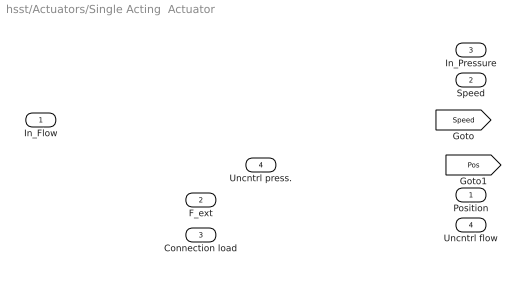
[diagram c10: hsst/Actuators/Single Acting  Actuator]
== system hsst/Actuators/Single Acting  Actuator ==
  In_Flow : Inport  Port=1  PortWidth=-1  SampleTime=-1  DataType=auto
  F_ext : Inport  Port=2  PortWidth=-1  SampleTime=-1  DataType=auto
  Connection load : Inport  Port=3  PortWidth=-1  SampleTime=-1  DataType=auto
  Uncntrl press. : Inport  Port=4  PortWidth=-1  SampleTime=-1  DataType=auto
  Position : Outport  Port=1
  Speed : Outport  Port=2
  In_Pressure : Outport  Port=3
  Uncntrl flow : Outport  Port=4
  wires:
  Uncntrl press./1 -> ?
  In_Flow/1 -> ?
  ? -> [Speed], Speed/1
  ? -> Position/1, [Pos]
  ? -> Uncntrl flow/1

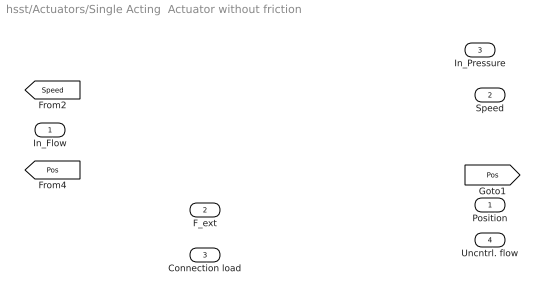
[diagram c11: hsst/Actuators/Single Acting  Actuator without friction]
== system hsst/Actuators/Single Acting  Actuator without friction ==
  In_Flow : Inport  Port=1  PortWidth=-1  SampleTime=-1  DataType=auto
  F_ext : Inport  Port=2  PortWidth=-1  SampleTime=-1  DataType=auto
  Connection load : Inport  Port=3  PortWidth=-1  SampleTime=-1  DataType=auto
  Position : Outport  Port=1
  Speed : Outport  Port=2
  In_Pressure : Outport  Port=3
  Uncntrl. flow : Outport  Port=4
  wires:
  In_Flow/1 -> ?
  [Speed] -> ?
  [Pos] -> ?
  F_ext/1 -> ?
  Connection load/1 -> ?

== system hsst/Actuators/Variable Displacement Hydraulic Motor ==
  In_Flows : Inport  Port=1  PortWidth=-1  SampleTime=-1  DataType=auto
  T_ext : Inport  Port=2  PortWidth=-1  SampleTime=-1  DataType=auto
  System_Pressures : Inport  Port=3  PortWidth=-1  SampleTime=-1  DataType=auto
  Connection Torque : Inport  Port=4  PortWidth=-1  SampleTime=-1  DataType=auto
  Position : Outport  Port=1
  Speed : Outport  Port=2
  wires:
  In_Flows/1 -> ?
  ? -> Position/1
  Connection Torque/1 -> ?
  T_ext/1 -> ?
  ? -> [Speed], Speed/1

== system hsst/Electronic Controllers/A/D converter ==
  In1 : Inport  Port=1  PortWidth=-1  SampleTime=-1  DataType=auto
  Out1 : Outport  Port=1  InitialOutput=0
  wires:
  ? -> Out1/1
  In1/1 -> ?

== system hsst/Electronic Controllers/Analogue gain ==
  Feedback : Inport  Port=1  PortWidth=-1  SampleTime=-1  DataType=auto
  Demand : Inport  Port=2  PortWidth=-1  SampleTime=-1  DataType=auto
  Pressures : Inport  Port=3  PortWidth=-1  SampleTime=-1  DataType=auto
  Current : Outport  Port=1
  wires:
  Pressures/1 -> ?

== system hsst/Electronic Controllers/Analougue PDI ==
  Feedback : Inport  Port=1  PortWidth=-1  SampleTime=-1  DataType=auto
  Demand : Inport  Port=2  PortWidth=-1  SampleTime=-1  DataType=auto
  Pressures : Inport  Port=3  PortWidth=-1  SampleTime=-1  DataType=auto
  Current : Outport  Port=1
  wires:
  ? -> Current/1
  Pressures/1 -> ?

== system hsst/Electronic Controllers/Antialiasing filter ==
  In Fdbk : Inport  Port=1  PortWidth=-1  SampleTime=-1  DataType=auto
  Out Fdbk : Outport  Port=1  InitialOutput=0
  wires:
  In Fdbk/1 -> ?
  ? -> Out Fdbk/1

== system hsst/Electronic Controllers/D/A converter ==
  In1 : Inport  Port=1  PortWidth=-1  SampleTime=-1  DataType=auto
  Out1 : Outport  Port=1  InitialOutput=0
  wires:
  ? -> Out1/1
  In1/1 -> ?

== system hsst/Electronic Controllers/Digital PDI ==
  Feedback : Inport  Port=1  PortWidth=-1  SampleTime=-1  DataType=auto
  Demand : Inport  Port=2  PortWidth=-1  SampleTime=-1  DataType=auto
  Pressures : Inport  Port=3  PortWidth=-1  SampleTime=-1  DataType=auto
  Current : Outport  Port=1
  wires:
  Pressures/1 -> ?
  Feedback/1 -> ?
  ? -> Current/1

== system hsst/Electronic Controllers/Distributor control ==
  Feedback : Inport  Port=1  PortWidth=-1  SampleTime=-1  DataType=auto
  Demand : Inport  Port=2  PortWidth=-1  SampleTime=-1  DataType=auto
  Pressures : Inport  Port=3  PortWidth=-1  SampleTime=-1  DataType=auto
  Current : Outport  Port=1
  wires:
  Pressures/1 -> ?

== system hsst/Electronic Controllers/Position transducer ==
  Position : Inport  Port=1  PortWidth=-1  SampleTime=-1  DataType=auto
  "Feedback " : Outport  Port=1  InitialOutput=0
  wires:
  Position/1 -> ?
  ? -> "Feedback "/1

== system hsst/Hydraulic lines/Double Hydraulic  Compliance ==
  In_Flows : Inport  Port=1  PortWidth=-1  SampleTime=-1  DataType=auto
  Out_Flows : Inport  Port=2  PortWidth=-1  SampleTime=-1  DataType=auto
  Out_Pressures : Outport  Port=1
  In_Pressures : Outport  Port=2
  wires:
  In_Flows/1 -> ?
  Out_Flows/1 -> ?

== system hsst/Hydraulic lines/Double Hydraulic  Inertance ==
  In_Pressures : Inport  Port=1  PortWidth=-1  SampleTime=-1  DataType=auto
  Out_Pressures : Inport  Port=2  PortWidth=-1  SampleTime=-1  DataType=auto
  Out_Flows : Outport  Port=1
  In_Flows : Outport  Port=2
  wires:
  In_Pressures/1 -> ?
  Out_Pressures/1 -> ?

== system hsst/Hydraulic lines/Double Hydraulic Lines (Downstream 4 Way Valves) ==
  In_Flows : Inport  Port=1  PortWidth=-1  SampleTime=-1  DataType=auto
  Out_Pressures : Inport  Port=2  PortWidth=-1  SampleTime=-1  DataType=auto
  Terminator : Terminator
  Out_Flows : Outport  Port=1
  In_Pressures : Outport  Port=2
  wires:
  ? -> Terminator/1
  ? -> Out_Flows/1

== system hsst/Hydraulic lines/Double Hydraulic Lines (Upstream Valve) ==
  Out_Flows : Inport  Port=1  PortWidth=-1  SampleTime=-1  DataType=auto
  In_Pressures : Inport  Port=2  PortWidth=-1  SampleTime=-1  DataType=auto
  Out_Pressures : Outport  Port=1
  In_Flows : Outport  Port=2
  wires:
  ? -> In_Flows/1
  ? -> ?
  In_Pressures/1 -> ?
  Out_Flows/1 -> ?

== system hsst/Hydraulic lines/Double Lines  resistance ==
  In_Pressures : Inport  Port=1  PortWidth=-1  SampleTime=-1  DataType=auto
  Out_Pressures : Inport  Port=2  PortWidth=-1  SampleTime=-1  DataType=auto
  In_Flows : Outport  Port=1  InitialOutput=0
  Out_flows : Outport  Port=2  InitialOutput=0
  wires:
  In_Pressures/1 -> ?
  Out_Pressures/1 -> ?

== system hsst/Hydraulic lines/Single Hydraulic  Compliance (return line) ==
  In_Flow : Inport  Port=1  PortWidth=-1  SampleTime=-1  DataType=auto
  Out_Flow : Inport  Port=2  PortWidth=-1  SampleTime=-1  DataType=auto
  Out_Pressure : Outport  Port=1
  In_Pressure : Outport  Port=2

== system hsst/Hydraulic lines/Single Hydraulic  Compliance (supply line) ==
  In_Flow : Inport  Port=1  PortWidth=-1  SampleTime=-1  DataType=auto
  Out_Flow : Inport  Port=2  PortWidth=-1  SampleTime=-1  DataType=auto
  Out_Pressure : Outport  Port=1
  In_Pressure : Outport  Port=2

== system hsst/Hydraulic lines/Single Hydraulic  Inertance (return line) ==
  In_Pressure : Inport  Port=1  PortWidth=-1  SampleTime=-1  DataType=auto
  Out_Pressure : Inport  Port=2  PortWidth=-1  SampleTime=-1  DataType=auto
  Out_Flow : Outport  Port=1
  In_Flow : Outport  Port=2

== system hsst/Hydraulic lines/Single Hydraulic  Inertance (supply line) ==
  In_Pressure : Inport  Port=1  PortWidth=-1  SampleTime=-1  DataType=auto
  Out_Pressure : Inport  Port=2  PortWidth=-1  SampleTime=-1  DataType=auto
  Out_Flow : Outport  Port=1
  In_Flow : Outport  Port=2

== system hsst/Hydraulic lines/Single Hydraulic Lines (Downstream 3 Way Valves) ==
  In_Flow : Inport  Port=1  PortWidth=-1  SampleTime=-1  DataType=auto
  Out_Pressure : Inport  Port=2  PortWidth=-1  SampleTime=-1  DataType=auto
  Terminator : Terminator
  Out_Flow : Outport  Port=1
  In_Pressure : Outport  Port=2
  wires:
  ? -> Terminator/1
  ? -> In_Pressure/1
  ? -> ?
  ? -> Out_Flow/1
  Out_Pressure/1 -> ?
  In_Flow/1 -> ?

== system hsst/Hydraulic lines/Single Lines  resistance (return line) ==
  In_Pressures : Inport  Port=1  PortWidth=-1  SampleTime=-1  DataType=auto
  Out_Pressures : Inport  Port=2  PortWidth=-1  SampleTime=-1  DataType=auto
  In_Flows : Outport  Port=1  InitialOutput=0
  Out_flows : Outport  Port=2  InitialOutput=0

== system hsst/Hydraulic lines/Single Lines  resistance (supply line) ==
  In_Pressures : Inport  Port=1  PortWidth=-1  SampleTime=-1  DataType=auto
  Out_Pressures : Inport  Port=2  PortWidth=-1  SampleTime=-1  DataType=auto
  In_Flows : Outport  Port=1  InitialOutput=0
  Out_flows : Outport  Port=2  InitialOutput=0

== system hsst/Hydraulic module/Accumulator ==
  Pump flow : Inport  Port=1  PortWidth=-1  SampleTime=-1  DataType=auto
  Out_Flow : Inport  Port=2  PortWidth=-1  SampleTime=-1  DataType=auto
  Relief flow : Inport  Port=3  PortWidth=-1  SampleTime=-1  DataType=auto
  Single acting act. unctrl. flow : Inport  Port=4  PortWidth=-1  SampleTime=-1  DataType=auto
  Out_Pressures : Outport  Port=1
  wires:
  Relief flow/1 -> ?
  Out_Flow/1 -> ?
  ? -> Out_Pressures/1

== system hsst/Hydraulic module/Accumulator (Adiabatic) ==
  Pump flow : Inport  Port=1  PortWidth=-1  SampleTime=-1  DataType=auto
  Out_Flow : Inport  Port=2  PortWidth=-1  SampleTime=-1  DataType=auto
  Relief flow : Inport  Port=3  PortWidth=-1  SampleTime=-1  DataType=auto
  Single acting act. unctrl. flow : Inport  Port=4  PortWidth=-1  SampleTime=-1  DataType=auto
  Out_Pressures : Outport  Port=1
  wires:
  ? -> Out_Pressures/1
  Out_Flow/1 -> ?

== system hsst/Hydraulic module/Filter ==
  In_Pressures : Inport  Port=1  PortWidth=-1  SampleTime=-1  DataType=auto
  Pump flow : Inport  Port=2  PortWidth=-1  SampleTime=-1  DataType=auto
  Out_Pressures : Outport  Port=1  InitialOutput=0
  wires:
  In_Pressures/1 -> ?
  Pump flow/1 -> ?
  ? -> Out_Pressures/1

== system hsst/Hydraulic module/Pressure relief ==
  In_Pressures : Inport  Port=1  PortWidth=-1  SampleTime=-1  DataType=auto
  Relief flow : Outport  Port=1

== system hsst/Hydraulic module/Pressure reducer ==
  In_Pressures : Inport  Port=1  PortWidth=-1  SampleTime=-1  DataType=auto
  Out_flows : Inport  Port=2  PortWidth=-1  SampleTime=-1  DataType=auto
  Reduceed pressures : Outport  Port=1  InitialOutput=0
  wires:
  Out_flows/1 -> ?
  In_Pressures/1 -> ?
  ? -> Reduceed pressures/1

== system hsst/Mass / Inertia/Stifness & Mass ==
  "Position " : Inport  Port=1  PortWidth=-1  SampleTime=-1  DataType=auto
  "Speed " : Inport  Port=2  PortWidth=-1  SampleTime=-1  DataType=auto
  F_ext2 : Inport  Port=3  PortWidth=-1  SampleTime=-1  DataType=auto
  Product5 : Product  Inputs=2  SaturateOnIntegerOverflow=on
  Position 2 : Outport  Port=1  InitialOutput=0
  Connection Load : Outport  Port=2  InitialOutput=0
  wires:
  "Speed "/1 -> ?
  F_ext2/1 -> ?
  ? -> Connection Load/1
  Product5/1 -> Position 2/1
  ? -> Product5/2

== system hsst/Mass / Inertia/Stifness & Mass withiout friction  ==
  "Position " : Inport  Port=1  PortWidth=-1  SampleTime=-1  DataType=auto
  "Speed " : Inport  Port=2  PortWidth=-1  SampleTime=-1  DataType=auto
  F_ext2 : Inport  Port=3  PortWidth=-1  SampleTime=-1  DataType=auto
  Position 2 : Outport  Port=1  InitialOutput=0
  Connection Load : Outport  Port=2  InitialOutput=0
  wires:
  ? -> Position 2/1
  "Position "/1 -> ?
  ? -> Connection Load/1
  F_ext2/1 -> ?
  "Speed "/1 -> ?

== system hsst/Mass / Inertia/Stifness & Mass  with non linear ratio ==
  "Position " : Inport  Port=1  PortWidth=-1  SampleTime=-1  DataType=auto
  "Speed " : Inport  Port=2  PortWidth=-1  SampleTime=-1  DataType=auto
  F_ext2 : Inport  Port=3  PortWidth=-1  SampleTime=-1  DataType=auto
  Position 2 : Outport  Port=1  InitialOutput=0
  Connection Load : Outport  Port=2  InitialOutput=0
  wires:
  ? -> Position 2/1
  F_ext2/1 -> ?
  "Speed "/1 -> ?
  ? -> Connection Load/1
  "Position "/1 -> ?

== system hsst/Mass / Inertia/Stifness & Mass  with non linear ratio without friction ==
  "Position " : Inport  Port=1  PortWidth=-1  SampleTime=-1  DataType=auto
  "Speed " : Inport  Port=2  PortWidth=-1  SampleTime=-1  DataType=auto
  F_ext2 : Inport  Port=3  PortWidth=-1  SampleTime=-1  DataType=auto
  Position 2 : Outport  Port=1  InitialOutput=0
  Connection Load : Outport  Port=2  InitialOutput=0
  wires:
  ? -> Connection Load/1
  "Speed "/1 -> ?
  F_ext2/1 -> ?
  ? -> Position 2/1

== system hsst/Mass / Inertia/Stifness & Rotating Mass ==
  "Position " : Inport  Port=1  PortWidth=-1  SampleTime=-1  DataType=auto
  "Speed " : Inport  Port=2  PortWidth=-1  SampleTime=-1  DataType=auto
  T_ext2 : Inport  Port=3  PortWidth=-1  SampleTime=-1  DataType=auto
  Product5 : Product  Inputs=2  SaturateOnIntegerOverflow=on
  Position 2 : Outport  Port=1  InitialOutput=0
  Connection Torque : Outport  Port=2  InitialOutput=0
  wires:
  "Speed "/1 -> ?
  T_ext2/1 -> ?
  Product5/1 -> Position 2/1

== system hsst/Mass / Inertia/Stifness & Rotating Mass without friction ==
  "Position " : Inport  Port=1  PortWidth=-1  SampleTime=-1  DataType=auto
  "Speed " : Inport  Port=2  PortWidth=-1  SampleTime=-1  DataType=auto
  T_ext2 : Inport  Port=3  PortWidth=-1  SampleTime=-1  DataType=auto
  Position 2 : Outport  Port=1  InitialOutput=0
  Connection Torque : Outport  Port=2  InitialOutput=0
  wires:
  ? -> Position 2/1
  ? -> Connection Torque/1
  T_ext2/1 -> ?
  "Speed "/1 -> ?

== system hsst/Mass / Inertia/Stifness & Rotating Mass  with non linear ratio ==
  "Position " : Inport  Port=1  PortWidth=-1  SampleTime=-1  DataType=auto
  "Speed " : Inport  Port=2  PortWidth=-1  SampleTime=-1  DataType=auto
  F_ext2 : Inport  Port=3  PortWidth=-1  SampleTime=-1  DataType=auto
  Product5 : Product  Inputs=2  SaturateOnIntegerOverflow=on
  Position 2 : Outport  Port=1  InitialOutput=0
  Connection Load : Outport  Port=2  InitialOutput=0
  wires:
  ? -> Connection Load/1
  "Speed "/1 -> ?
  F_ext2/1 -> ?
  Product5/1 -> Position 2/1
  "Position "/1 -> ?
  ? -> Product5/2

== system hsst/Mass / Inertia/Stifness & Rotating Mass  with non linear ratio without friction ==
  "Position " : Inport  Port=1  PortWidth=-1  SampleTime=-1  DataType=auto
  "Speed " : Inport  Port=2  PortWidth=-1  SampleTime=-1  DataType=auto
  F_ext2 : Inport  Port=3  PortWidth=-1  SampleTime=-1  DataType=auto
  Position 2 : Outport  Port=1  InitialOutput=0
  Connection Load : Outport  Port=2  InitialOutput=0
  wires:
  ? -> Position 2/1
  F_ext2/1 -> ?
  "Speed "/1 -> ?
  ? -> Connection Load/1

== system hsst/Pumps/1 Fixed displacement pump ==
  Angular speed : Inport  Port=1  PortWidth=-1  SampleTime=-1  DataType=auto
  Pump flow : Outport  Port=1
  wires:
  Angular speed/1 -> ?

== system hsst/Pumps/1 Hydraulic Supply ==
  Out_Flow : Inport  Port=1  PortWidth=-1  SampleTime=-1  DataType=auto
  Pressures : Outport  Port=1

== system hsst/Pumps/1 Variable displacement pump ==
  Angular speed : Inport  Port=1  PortWidth=-1  SampleTime=-1  DataType=auto
  Pressure : Inport  Port=2  PortWidth=-1  SampleTime=-1  DataType=auto
  Pump flow : Outport  Port=1
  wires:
  Pressure/1 -> ?

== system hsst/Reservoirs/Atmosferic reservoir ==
  Out _Flows : Inport  Port=1  PortWidth=-1  SampleTime=-1  DataType=auto
  Pump flow : Inport  Port=2  PortWidth=-1  SampleTime=-1  DataType=auto
  Relief flow : Inport  Port=3  PortWidth=-1  SampleTime=-1  DataType=auto
  Single acting act. unctrl. flow : Inport  Port=4  PortWidth=-1  SampleTime=-1  DataType=auto
  Reservoir volume : Outport  Port=1
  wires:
  ? -> Reservoir volume/1

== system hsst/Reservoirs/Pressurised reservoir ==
  Out _Flows : Inport  Port=1  PortWidth=-1  SampleTime=-1  DataType=auto
  Pump flow : Inport  Port=2  PortWidth=-1  SampleTime=-1  DataType=auto
  Relief flow : Inport  Port=3  PortWidth=-1  SampleTime=-1  DataType=auto
  Pressures : Inport  Port=4  PortWidth=-1  SampleTime=-1  DataType=auto
  Single acting act. unctrl. flow : Inport  Port=5  PortWidth=-1  SampleTime=-1  DataType=auto
  Reservoir volume : Outport  Port=1
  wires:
  Out _Flows/1 -> ?
  Pressures/1 -> ?
  ? -> [p_res]

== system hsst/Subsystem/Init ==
  Subsystem : Subsystem

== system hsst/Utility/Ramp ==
  Clock : Clock
  Constant : Constant  Value=start
  Constant1 : Constant  Value=X0
  Product : Product  Inputs=2  SaturateOnIntegerOverflow=on
  Step : Step  Time=start  Before=0  After=slope  SampleTime=0
  Sum : Sum  Inputs=|+-  SaturateOnIntegerOverflow=on
  Sum1 : Sum  Inputs=|++  SaturateOnIntegerOverflow=on
  Out1 : Outport  Port=1
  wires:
  Clock/1 -> Sum/1
  Constant/1 -> Sum/2
  Sum/1 -> Product/2
  Sum1/1 -> Out1/1
  Constant1/1 -> Sum1/2
  Product/1 -> Sum1/1
  Step/1 -> Product/1

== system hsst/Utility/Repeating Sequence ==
  Clock : Clock
  Fcn1 : Fcn  Expr=rem(u[1],period)
  Look-Up Table : Lookup  InputValues=rep_seq_t  OutputValues=rep_seq_y
  Out1 : Outport  Port=1
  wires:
  Look-Up Table/1 -> Out1/1
  Clock/1 -> Fcn1/1
  Fcn1/1 -> Look-Up Table/1

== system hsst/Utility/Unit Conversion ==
  Input : Inport  Port=1  PortWidth=-1  SampleTime=-1  DataType=auto
  Gain : Gain  Gain=gain  SaturateOnIntegerOverflow=on
  Out1 : Outport  Port=1
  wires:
  Input/1 -> Gain/1
  Gain/1 -> Out1/1

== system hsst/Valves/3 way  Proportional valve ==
  note: Servovalve Model
  Curr : Inport  Port=1  PortWidth=-1  SampleTime=-1  DataType=auto
  In_Pressures : Inport  Port=2  PortWidth=-1  SampleTime=-1  DataType=auto
  Out_Pressure : Inport  Port=3  PortWidth=-1  SampleTime=-1  DataType=auto
  In_Flows : Outport  Port=1  InitialOutput=0
  Out_Flow : Outport  Port=2  InitialOutput=0
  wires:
  ? -> Out_Flow/1
  Curr/1 -> ?
  ? -> In_Flows/1
